(* Logix 5000 AddOnInstructionDefinition export EH_Smartec_CLD18_IOL; software revision 38.00 *)

TYPE EH_CommAOI_Data :
STRUCT
   Device_Comm_Error : BOOL;
   CommSuccess : BOOL;
   CommFailed : BOOL;
   CommTimeOut : BOOL;
   StateDone : BOOL;
   NewState : BOOL;
   OldState : SINT;
   PortSize : SINT;
   DevicePort : SINT;
   MaxState : SINT;
   State : SINT;
   VendorID : INT;
   DeviceID : DINT;
   CyclicData : INT[16];
   AcyclicData : DINT[8];
   ReplayIndex : INT;
   AOI_Diagnostic : DINT;
   ConnectionStatus : DINT;
   OutputData : INT[16];
END_STRUCT
END_TYPE

ADD_ON_INSTRUCTION EH_Smartec_CLD18_IOL   (* revision 1.0, vendor Endress+Hauser *)
// Smartec CLD18 Rev 1 IO-Link
VAR_IN_OUT
   DataToSend : INT[10]; {required}
   CommAOIBusy : DINT; {required}
   ActiveComPort : DINT; {required}
   DeviceAOISendRequest : DINT; {required}
   CommError : INT; {required}
   DeviceData : EH_CommAOI_Data; {required}
END_VAR
VAR_OUTPUT
   qVendor_ID : DINT; {access Read Only, visible}
   qDevice_ID : DINT; {access Read Only, visible}
END_VAR
VAR_INPUT
   iExecuteRisingEdge : BOOL; {visible}
   iSetSimulation : BOOL; {visible}
   iSetSimulationConductivity : REAL; {visible}
   iSetSimulationTemp : REAL; {visible}
   iParameterSet : SINT; {visible}
END_VAR
VAR_OUTPUT
   qConductivity : REAL; {visible}
   qTemperature : REAL; {visible}
   qCondensedStatus : USINT; {visible}
   qSSC1_1 : BOOL; {access Read Only, visible}
   qSSC1_2 : BOOL; {visible}
   qSSC2_1 : BOOL; {visible}
   qSSC2_2 : BOOL; {visible}
   qActiveParameterSet : BOOL; {visible}
   qSimulationActive : BOOL; {access Read Only, visible}
   qAOI_Diagnostic : DINT; {access Read Only, visible}
END_VAR
VAR_IN_OUT
   qActual_Diagnostics_String : STRING; {required}
END_VAR
VAR_OUTPUT
   qActual_Diagnostics_Code : DINT; {access Read Only, visible}
END_VAR
VAR_IN_OUT
   qLast_Diagnostics_String : STRING; {required}
END_VAR
VAR_OUTPUT
   qLast_Diagnostics_Code : DINT; {visible}
   qCommunicationBusy : DINT; {access Read Only, visible}
   qCommError : DINT; {access Read Only, visible}
   qDeviceConnectionError : BOOL; {access Read Only, visible}
END_VAR
VAR_INPUT
   DeviceID1 : DINT;
   qDevice_ID_select : INT;
END_VAR
VAR
   Calc_DID : DINT; {access None}
   Calc_VID : DINT; {access None}
   Cond_DINT : DINT; {access None}
   Temp_DINT : DINT; {access None}
   Calc_Cond : DINT; {access None}
   Cald_Temp : DINT; {access None}
   Calc_Temp : DINT; {access None}
   Calc_CondenStatus : DINT; {access None}
   CMD_Index : INT; {access None}
   CMD_Subindex : INT; {access None}
   CMD_ByteLength : INT; {access None}
   StateMin : INT; {access None}
   Trigger : BOOL; {access None}
   CMD_Rd : BOOL; {access None}
   CMD_Wr : BOOL; {access None}
   SimulationDINT : DINT; {access None}
   InputByteLength : DINT; {access None}
   oldCondStatus : USINT; {access None}
   ActiveAOI : BOOL; {access None}
   AOI_Prio : BOOL; {access None}
   firstTimeDone : BOOL; {access None}
   CondStatusChanged : BOOL; {access None}
   DeviceID : DINT; {access None}
   FALSE : BOOL; {access None}
   TRUE : BOOL := 1; {access None}
END_VAR

ROUTINE Logic   (* structured text *)
// CLD18 Communication via AL1323
   // =======================================================================
   // Endress+Hauser Digital Solutions
   // ©Copyright (2024) All Rights Reserved
   // =======================================================================
   // Name:                EH_Smartec_CLD18_IOL
   // Version:             1.0
   // Datum:               11.2025
   // Library:             01.01.00
   // Engineering:         Studio5000 V38.00.00
   // Author:              EH
   // =======================================================================
   
   
   qAOI_Diagnostic := DeviceData.AOI_Diagnostic;
   qCommunicationBusy := CommAOIBusy;
   DeviceID1 := 131329;
   StateMin := 0;
   DeviceData.MaxState := 8;
   
   if DeviceData.DevicePort = 0 or DeviceData.DeviceID <> DeviceID1 or DeviceData.ConnectionStatus <> 1 then
   
   	qVendor_ID	:= 0;
   	qDevice_ID	:= 0;
   	qConductivity	:= 0;
   	qTemperature	:= 0;
   	qCondensedStatus	:= 0;
   	qSSC1_1	:= 0;
   	qSSC1_2	:= 0;
   	qSSC2_1	:= 0;
   	qSSC2_2	:= 0;
   	qActiveParameterSet	:= 0;
   	qSimulationActive	:= 0;
   	qActual_Diagnostics_Code	:= 0;
   	qLast_Diagnostics_Code	:= 0;
   	qLast_Diagnostics_String	:= '';
   
   	if DeviceData.DevicePort = 0 then
   
   		qActual_Diagnostics_String	:= 'Device Port is Zero';
   		DeviceData.AOI_Diagnostic.1 := TRUE;
   
   	elsif DeviceData.ConnectionStatus <> 1 then
   
   		qActual_Diagnostics_String	:= 'No Device connected';
   		qDeviceConnectionError := TRUE;
   
   	elsif DeviceData.DeviceID <> DeviceID1 then
   
   		qActual_Diagnostics_String	:= 'Wrong DeviceID';
   		DeviceData.AOI_Diagnostic.2 := TRUE;
   		qVendor_ID := DeviceData.VendorID;
   		qDevice_ID := DeviceData.DeviceID;
   
   	end_if;
   
   else
   
   	if qActual_Diagnostics_Code = 0 then
   
   		qActual_Diagnostics_String	:= '--------';
   
   	end_if;
   
   	if qLast_Diagnostics_Code = 0 then
   
   		qLast_Diagnostics_String	:= '--------';
   
   	end_if;
   
   	DeviceData.AOI_Diagnostic.1 := FALSE;
   	qDeviceConnectionError := FALSE;
   	DeviceData.AOI_Diagnostic.2  := FALSE;
   
   end_if;
   
   
   if not DeviceData.AOI_Diagnostic.0
   	and not qDeviceConnectionError
   	and not DeviceData.AOI_Diagnostic.2
   	and DeviceData.DevicePort > 0 or ActiveAOI and qDeviceConnectionError then
   
   	//*********************************
   	//Vendor ID
   	//*********************************
   
   	qVendor_ID := DeviceData.VendorID;
   
   	//*********************************
   	//Device ID
   	//*********************************
   
   	qDevice_ID := DeviceData.DeviceID;
   
   	if DeviceData.DeviceID = DeviceID1 then
   
   		qDevice_ID_select :=1;
   
   	else
   
   		qDevice_ID_select := 0;
   
   	end_if;
   
   	case qDevice_ID_select of
   
   		1:
   
   		Calc_Cond 			:= 0+((DeviceData.DevicePort-1)*InputByteLength);  // Startwert 190 + Protnummer mal Datalength 32Byte
   		Calc_Temp 			:= 2+((DeviceData.DevicePort-1)*InputByteLength);  // Startwert 194 + Protnummer mal Datalength 32Byte
   		Calc_CondenStatus 	:= 4+((DeviceData.DevicePort-1)*InputByteLength); // Startwert 198 + Protnummer mal Datalength 32Byte
   
   		//*********************************
   		//Process Data Cond
   		//*********************************
   
   		Cond_DINT := DeviceData.CyclicData[Calc_Cond+1];
   		Cond_DINT.8 := DeviceData.CyclicData[Calc_Cond+1].8;
   		Cond_DINT.9 := DeviceData.CyclicData[Calc_Cond+1].9;
   		Cond_DINT.10 := DeviceData.CyclicData[Calc_Cond+1].10;
   		Cond_DINT.11 := DeviceData.CyclicData[Calc_Cond+1].11;
   		Cond_DINT.12 := DeviceData.CyclicData[Calc_Cond+1].12;
   		Cond_DINT.13 := DeviceData.CyclicData[Calc_Cond+1].13;
   		Cond_DINT.14 := DeviceData.CyclicData[Calc_Cond+1].14;
   		Cond_DINT.15 := DeviceData.CyclicData[Calc_Cond+1].15;
   		Cond_DINT.16 := DeviceData.CyclicData[Calc_Cond].0;
   		Cond_DINT.17 := DeviceData.CyclicData[Calc_Cond].1;
   		Cond_DINT.18 := DeviceData.CyclicData[Calc_Cond].2;
   		Cond_DINT.19 := DeviceData.CyclicData[Calc_Cond].3;
   		Cond_DINT.20 := DeviceData.CyclicData[Calc_Cond].4;
   		Cond_DINT.21 := DeviceData.CyclicData[Calc_Cond].5;
   		Cond_DINT.22 := DeviceData.CyclicData[Calc_Cond].6;
   		Cond_DINT.23 := DeviceData.CyclicData[Calc_Cond].7;
   		Cond_DINT.24 := DeviceData.CyclicData[Calc_Cond].8;
   		Cond_DINT.25 := DeviceData.CyclicData[Calc_Cond].9;
   		Cond_DINT.26 := DeviceData.CyclicData[Calc_Cond].10;
   		Cond_DINT.27 := DeviceData.CyclicData[Calc_Cond].11;
   		Cond_DINT.28 := DeviceData.CyclicData[Calc_Cond].12;
   		Cond_DINT.29 := DeviceData.CyclicData[Calc_Cond].13;
   		Cond_DINT.30 := DeviceData.CyclicData[Calc_Cond].14;
   		Cond_DINT.31 := DeviceData.CyclicData[Calc_Cond].15;
   
   		COP(Cond_DINT,qConductivity,1);
   
   		//*********************************
   		//Process Data Temp
   		//*********************************
   
   		Temp_DINT := DeviceData.CyclicData[Calc_Temp+1];
   		Temp_DINT.8 := DeviceData.CyclicData[Calc_Temp+1].8;
   		Temp_DINT.9 := DeviceData.CyclicData[Calc_Temp+1].9;
   		Temp_DINT.10 := DeviceData.CyclicData[Calc_Temp+1].10;
   		Temp_DINT.11 := DeviceData.CyclicData[Calc_Temp+1].11;
   		Temp_DINT.12 := DeviceData.CyclicData[Calc_Temp+1].12;
   		Temp_DINT.13 := DeviceData.CyclicData[Calc_Temp+1].13;
   		Temp_DINT.14 := DeviceData.CyclicData[Calc_Temp+1].14;
   		Temp_DINT.15 := DeviceData.CyclicData[Calc_Temp+1].15;
   		Temp_DINT.16 := DeviceData.CyclicData[Calc_Temp].0;
   		Temp_DINT.17 := DeviceData.CyclicData[Calc_Temp].1;
   		Temp_DINT.18 := DeviceData.CyclicData[Calc_Temp].2;
   		Temp_DINT.19 := DeviceData.CyclicData[Calc_Temp].3;
   		Temp_DINT.20 := DeviceData.CyclicData[Calc_Temp].4;
   		Temp_DINT.21 := DeviceData.CyclicData[Calc_Temp].5;
   		Temp_DINT.22 := DeviceData.CyclicData[Calc_Temp].6;
   		Temp_DINT.23 := DeviceData.CyclicData[Calc_Temp].7;
   		Temp_DINT.24 := DeviceData.CyclicData[Calc_Temp].8;
   		Temp_DINT.25 := DeviceData.CyclicData[Calc_Temp].9;
   		Temp_DINT.26 := DeviceData.CyclicData[Calc_Temp].10;
   		Temp_DINT.27 := DeviceData.CyclicData[Calc_Temp].11;
   		Temp_DINT.28 := DeviceData.CyclicData[Calc_Temp].12;
   		Temp_DINT.29 := DeviceData.CyclicData[Calc_Temp].13;
   		Temp_DINT.30 := DeviceData.CyclicData[Calc_Temp].14;
   		Temp_DINT.31 := DeviceData.CyclicData[Calc_Temp].15;
   
   		COP(Temp_DINT,qTemperature,1);
   
   		//*********************************
   		// Cond Status
   		//*********************************
   
   		qCondensedStatus.0 := DeviceData.CyclicData[Calc_CondenStatus].8;
   		qCondensedStatus.1 := DeviceData.CyclicData[Calc_CondenStatus].9;
   		qCondensedStatus.2 := DeviceData.CyclicData[Calc_CondenStatus].10;
   		qCondensedStatus.3 := DeviceData.CyclicData[Calc_CondenStatus].11;
   		qCondensedStatus.4 := DeviceData.CyclicData[Calc_CondenStatus].12;
   		qCondensedStatus.5 := DeviceData.CyclicData[Calc_CondenStatus].13;
   		qCondensedStatus.6 := DeviceData.CyclicData[Calc_CondenStatus].14;
   		qCondensedStatus.7 := DeviceData.CyclicData[Calc_CondenStatus].15;
   
   		//*********************************
   		//SSC Outputs
   		//*********************************
   
   		qSSC1_1 := DeviceData.CyclicData[Calc_CondenStatus].0;
   		qSSC1_2 := DeviceData.CyclicData[Calc_CondenStatus].1;
   		qSSC2_1 := DeviceData.CyclicData[Calc_CondenStatus].2;
   		qSSC2_2 := DeviceData.CyclicData[Calc_CondenStatus].3;
   
   		//*********************************
   		//Active Parameter Set
   		//*********************************
   
   		qActiveParameterSet := DeviceData.CyclicData[Calc_CondenStatus].4;
   
   		//*********************************
   		//CondenstStatus
   		//*********************************
   
   		qCondensedStatus.0 := DeviceData.CyclicData[Calc_CondenStatus].8;
   		qCondensedStatus.1 := DeviceData.CyclicData[Calc_CondenStatus].9;
   		qCondensedStatus.2 := DeviceData.CyclicData[Calc_CondenStatus].10;
   		qCondensedStatus.3 := DeviceData.CyclicData[Calc_CondenStatus].11;
   		qCondensedStatus.4 := DeviceData.CyclicData[Calc_CondenStatus].12;
   		qCondensedStatus.5 := DeviceData.CyclicData[Calc_CondenStatus].13;
   		qCondensedStatus.6 := DeviceData.CyclicData[Calc_CondenStatus].14;
   		qCondensedStatus.7 := DeviceData.CyclicData[Calc_CondenStatus].15;
   
   	end_case;
   
   	if  oldCondStatus = qCondensedStatus then
   
   		CondStatusChanged := 1;
   
   	else
   
   		CondStatusChanged := 0;
   
   	end_if;
   
   	//*********************************
   	// Checking for CommBlockBusy
   	//*********************************
   
   	if iExecuteRisingEdge and DeviceData.State = 0 and not ActiveAOI then
   		DeviceAOISendRequest.[DeviceData.DevicePort] := 1;
   
   	end_if;
   
   	if not CondStatusChanged and not ActiveAOI then
   		DeviceAOISendRequest.[DeviceData.DevicePort] := 1;
   
   	end_if;
   
   	if ActiveComPort = DeviceData.DevicePort then
   
   		AOI_Prio :=1;
   	else
   
   		AOI_Prio := 0;
   	end_if;
   
   
   	if CommAOIBusy = 1 and iExecuteRisingEdge and DeviceData.State = 0 and AOI_Prio and not ActiveAOI then
   
   		ActiveAOI := 1;
   
   	end_if;
   
   	if CommAOIBusy = 1 and not CondStatusChanged and (DeviceData.State = 0 or DeviceData.State = DeviceData.MaxState) and AOI_Prio and not ActiveAOI then
   
   		ActiveAOI := 1;
   
   	end_if;
   
   
   
   	qCommunicationBusy := CommAOIBusy;
   	qAOI_Diagnostic :=DeviceData.AOI_Diagnostic;
   
   
   	if  ActiveAOI and qDeviceConnectionError then
   
   		DeviceData.State := DeviceData.MaxState;
   
   	end_if;
   
   	//*********************************
   	// State machine
   	//*********************************
   
   	if ActiveAOI or DeviceData.State = DeviceData.MaxState then
   
   	case DeviceData.State of
   
   		//*********************************
   		0: // Idle
   		//*********************************
   
   			// Initializing
   			Trigger := 0;
   			CMD_Index := 0;
   			CMD_Subindex := 0;
   			CMD_Wr := 0;
   			CMD_Rd := 0;
   			CMD_ByteLength := 0;
   
   			if DeviceData.DevicePort = ActiveComPort then
   					DeviceData.CommSuccess := 0;
   					DeviceData.CommTimeOut := 0;
   					DeviceData.NewState := 1;
   					DeviceData.StateDone := 0;
   			end_if;
   
   			// Wait for trigger
   			if iExecuteRisingEdge and ActiveComPort = DeviceData.DevicePort then
   
   				DeviceData.AOI_Diagnostic := 0;
   				DeviceData.State := DeviceData.State + 1;
   
   			end_if;
   
   			if not CondStatusChanged then
   
   				DeviceData.State := DeviceData.MaxState - 2;
   				oldCondStatus := qCondensedStatus;
   
   			end_if;
   
   		//*********************************
   		1: // Simulation
   		//*********************************
   
   		    CMD_Index := 101;
   		    CMD_Subindex := 0;
   		    CMD_Wr := 1;
   			CMD_Rd := 0;
   		    CMD_ByteLength := 2;
   			DataToSend[6]:= 0;
   			DataToSend[7]:= 0;
   
   			if DeviceData.NewState then
   
   				DeviceData.StateDone := 1;
   
   			end_if;
   
   		    if iSetSimulation then
   
   		       DataToSend[6].8 := 1;
   
   		    else
   
   		        DataToSend[6].8 := 0;
   
   		    end_if;
   
   		    Trigger := 1;
   
   			if  DeviceData.CommSuccess and DeviceData.ReplayIndex = CMD_Index then
   
   				Trigger := 0;
   				DeviceData.OldState := DeviceData.State;
   		        DeviceData.State := DeviceData.State + 1;
   				DeviceData.CommSuccess := 0;
   				DeviceData.AcyclicData[0] := 0;
   				DeviceData.NewState := 1;
   
   			 elsif DeviceData.CommTimeOut then
   
   				DeviceData.AOI_Diagnostic.[DeviceData.State+7] := 1;
   				DeviceData.OldState := DeviceData.State;
   		        DeviceData.State := DeviceData.State + 1;
   				DeviceData.CommTimeOut := 0;
   				DeviceData.AcyclicData[0] := 0;
   				DeviceData.NewState := 1;
   
   		    end_if;
   
   		//*********************************
   		2: // Simulation - Value Cond
   		//*********************************
   
   		    CMD_Index := 102;
   		    CMD_Subindex := 0;
   		    CMD_Wr := 1;
   			CMD_Rd := 0;
   		    CMD_ByteLength := 4;
   
   			if DeviceData.NewState then
   
   				DeviceData.StateDone := 1;
   
   			end_if;
   
   			COP(iSetSimulationConductivity,SimulationDINT,1); // Kopiert den Inhalt des Real in ein DINT Format. Dabei wird nicht der eigentliche Realwert kopiert.
   
   			DataToSend[6].0 :=  SimulationDINT.24;
   			DataToSend[6].1 :=  SimulationDINT.25;
   			DataToSend[6].2 :=  SimulationDINT.26;
   			DataToSend[6].3 :=  SimulationDINT.27;
   			DataToSend[6].4 :=  SimulationDINT.28;
   			DataToSend[6].5 :=  SimulationDINT.29;
   			DataToSend[6].6 :=  SimulationDINT.30;
   			DataToSend[6].7 :=  SimulationDINT.31;
   			DataToSend[6].8 :=  SimulationDINT.16;
   			DataToSend[6].9 :=  SimulationDINT.17;
   			DataToSend[6].10 := SimulationDINT.18;
   			DataToSend[6].11 := SimulationDINT.19;
   			DataToSend[6].12 := SimulationDINT.20;
   			DataToSend[6].13 := SimulationDINT.21;
   			DataToSend[6].14 := SimulationDINT.22;
   			DataToSend[6].15 := SimulationDINT.23;
   			DataToSend[7].0  := SimulationDINT.8;
   			DataToSend[7].1  := SimulationDINT.9;
   			DataToSend[7].2  := SimulationDINT.10;
   			DataToSend[7].3  := SimulationDINT.11;
   			DataToSend[7].4  := SimulationDINT.12;
   			DataToSend[7].5  := SimulationDINT.13;
   			DataToSend[7].6  := SimulationDINT.14;
   			DataToSend[7].7  := SimulationDINT.15;
   			DataToSend[7].8  := SimulationDINT.0;
   			DataToSend[7].9  := SimulationDINT.1;
   			DataToSend[7].10 := SimulationDINT.2;
   			DataToSend[7].11 := SimulationDINT.3;
   			DataToSend[7].12 := SimulationDINT.4;
   			DataToSend[7].13 := SimulationDINT.5;
   			DataToSend[7].14 := SimulationDINT.6;
   			DataToSend[7].15 := SimulationDINT.7;
   			Trigger := 1;
   
   			if  DeviceData.CommSuccess and DeviceData.ReplayIndex = CMD_Index then
   
   				Trigger := 0;
   				DeviceData.OldState := DeviceData.State;
   		        DeviceData.State := DeviceData.State + 1;
   				DeviceData.CommSuccess := 0;
   				DeviceData.AcyclicData[0] := 0;
   				DeviceData.NewState := 1;
   
   			 elsif DeviceData.CommTimeOut then
   
   				DeviceData.AOI_Diagnostic.[DeviceData.State+7] := 1;
   				DeviceData.OldState := DeviceData.State;
   		        DeviceData.State := DeviceData.State + 1;
   				DeviceData.CommTimeOut := 0;
   				DeviceData.AcyclicData[0] := 0;
   				DeviceData.NewState := 1;
   
   		    end_if;
   
   		//*********************************
   		3: // Simulation - Value Temp
   		//*********************************
   
   		    CMD_Index := 103;
   		    CMD_Subindex := 0;
   		    CMD_Wr := 1;
   			CMD_Rd := 0;
   		    CMD_ByteLength := 4;
   
   			if DeviceData.NewState then
   
   				DeviceData.StateDone := 1;
   
   			end_if;
   
   			COP(iSetSimulationTemp,SimulationDINT,1); // Kopiert den Inhalt des Real in ein DINT Format. Dabei wird nicht der eigentliche Realwert kopiert.
   
   			DataToSend[6].0 :=  SimulationDINT.24;
   			DataToSend[6].1 :=  SimulationDINT.25;
   			DataToSend[6].2 :=  SimulationDINT.26;
   			DataToSend[6].3 :=  SimulationDINT.27;
   			DataToSend[6].4 :=  SimulationDINT.28;
   			DataToSend[6].5 :=  SimulationDINT.29;
   			DataToSend[6].6 :=  SimulationDINT.30;
   			DataToSend[6].7 :=  SimulationDINT.31;
   			DataToSend[6].8 :=  SimulationDINT.16;
   			DataToSend[6].9 :=  SimulationDINT.17;
   			DataToSend[6].10 := SimulationDINT.18;
   			DataToSend[6].11 := SimulationDINT.19;
   			DataToSend[6].12 := SimulationDINT.20;
   			DataToSend[6].13 := SimulationDINT.21;
   			DataToSend[6].14 := SimulationDINT.22;
   			DataToSend[6].15 := SimulationDINT.23;
   			DataToSend[7].0  := SimulationDINT.8;
   			DataToSend[7].1  := SimulationDINT.9;
   			DataToSend[7].2  := SimulationDINT.10;
   			DataToSend[7].3  := SimulationDINT.11;
   			DataToSend[7].4  := SimulationDINT.12;
   			DataToSend[7].5  := SimulationDINT.13;
   			DataToSend[7].6  := SimulationDINT.14;
   			DataToSend[7].7  := SimulationDINT.15;
   			DataToSend[7].8  := SimulationDINT.0;
   			DataToSend[7].9  := SimulationDINT.1;
   			DataToSend[7].10 := SimulationDINT.2;
   			DataToSend[7].11 := SimulationDINT.3;
   			DataToSend[7].12 := SimulationDINT.4;
   			DataToSend[7].13 := SimulationDINT.5;
   			DataToSend[7].14 := SimulationDINT.6;
   			DataToSend[7].15 := SimulationDINT.7;
   			Trigger := 1;
   
   			if  DeviceData.CommSuccess and DeviceData.ReplayIndex = CMD_Index then
   
   				Trigger := 0;
   				DeviceData.OldState := DeviceData.State;
   		        DeviceData.State := DeviceData.State + 1;
   				DeviceData.CommSuccess := 0;
   				DeviceData.AcyclicData[0] := 0;
   				DeviceData.NewState := 1;
   
   			 elsif DeviceData.CommTimeOut then
   
   				DeviceData.AOI_Diagnostic.[DeviceData.State+7] := 1;
   				DeviceData.OldState := DeviceData.State;
   		        DeviceData.State := DeviceData.State + 1;
   				DeviceData.CommTimeOut := 0;
   				DeviceData.AcyclicData[0] := 0;
   				DeviceData.NewState := 1;
   
   		    end_if;
   
   		//*********************************
   		4: // Simulation - Value ParameterSet
   		//*********************************
   
   		    CMD_Index := 112;
   		    CMD_Subindex := 0;
   		    CMD_Wr := 1;
   			CMD_Rd := 0;
   		    CMD_ByteLength := 1;
   			DataToSend[6]:= 0;
   			DataToSend[7]:= 0;
   			Trigger := 1;
   
   			if DeviceData.NewState then
   
   				DeviceData.StateDone := 1;
   
   			end_if;
   
   			if iParameterSet = 1 then
   
   		       DataToSend[6] := 0;
   
   		    elsif iParameterSet = 2 then
   
   		        DataToSend[6] := 1;
   
   		    end_if;
   
   			if  DeviceData.CommSuccess and DeviceData.ReplayIndex = CMD_Index then
   
   				Trigger := 0;
   				DeviceData.OldState := DeviceData.State;
   		        DeviceData.State := DeviceData.State + 1;
   				DeviceData.CommSuccess := 0;
   				DeviceData.AcyclicData[0] := 0;
   				DeviceData.NewState := 1;
   
   			 elsif DeviceData.CommTimeOut then
   
   				DeviceData.AOI_Diagnostic.[DeviceData.State+7] := 1;
   				DeviceData.OldState := DeviceData.State;
   		        DeviceData.State := DeviceData.State + 1;
   				DeviceData.CommTimeOut := 0;
   				DeviceData.AcyclicData[0] := 0;
   				DeviceData.NewState := 1;
   
   		    end_if;
   
   		//*********************************
   		5: // Simulation - SimulationActive
   		//*********************************
   
   		    CMD_Index := 101;
   		    CMD_Subindex := 0;
   		    CMD_Wr := 0;
   			CMD_Rd := 1;
   		    CMD_ByteLength := 0;
   			Trigger := 1;
   
   			if DeviceData.NewState then
   
   				DeviceData.StateDone := 1;
   
   			end_if;
   
   			if  DeviceData.CommSuccess and DeviceData.ReplayIndex = CMD_Index then
   
   				qSimulationActive := DeviceData.AcyclicData[0].0;
   
   				Trigger := 0;
   				DeviceData.OldState := DeviceData.State;
   		        DeviceData.State := DeviceData.State + 1;
   				DeviceData.CommSuccess := 0;
   				DeviceData.AcyclicData[0] := 0;
   				DeviceData.NewState := 1;
   
   			 elsif DeviceData.CommTimeOut then
   
   				DeviceData.AOI_Diagnostic.[DeviceData.State+7] := 1;
   				DeviceData.OldState := DeviceData.State;
   		        DeviceData.State := DeviceData.State + 1;
   				DeviceData.CommTimeOut := 0;
   				DeviceData.AcyclicData[0] := 0;
   				DeviceData.NewState := 1;
   
   		    end_if;
   
   		//*********************************
   		6: // Actual Diagnostic
   		//*********************************
   
   		    CMD_Index := 260;
   		    CMD_Subindex := 0;
   		    CMD_Wr := 0;
   			CMD_Rd := 1;
   		    Trigger := 1;
   			if DeviceData.NewState then
   			DeviceData.StateDone := 1;
   			end_if;
   
   			if  DeviceData.CommSuccess and DeviceData.ReplayIndex = CMD_Index then
   
   				qActual_Diagnostics_Code	:= DeviceData.AcyclicData[0];
   
   				case qActual_Diagnostics_Code of
   
   		            0:
   		                qActual_Diagnostics_String := 'System ok';
   		            1:
   		                qActual_Diagnostics_String := 'no communication';
   		            22:
   		                qActual_Diagnostics_String := 'F022 Temperature sensor is defective';
   		            61:
   		                qActual_Diagnostics_String := 'F061 Sensor electronics defective';
   		            100:
   		                qActual_Diagnostics_String := 'F100 Sensor not communicating, not connected';
   		            130:
   		                qActual_Diagnostics_String := 'F130 Sensor check, no conductivity displayed';
   		            152:
   		                qActual_Diagnostics_String := 'F152 Sensor data No calibration data available';
   		            241:
   		                qActual_Diagnostics_String := 'F241 Unspecific software error';
   		            243:
   		                qActual_Diagnostics_String := 'F243 Unspecific hardware error';
   		            419:
   		                qActual_Diagnostics_String := 'F419 Back to box command is executed';
   		            904:
   		                qActual_Diagnostics_String := 'F904 Process check system alarm';
   		            107:
   		                qActual_Diagnostics_String := 'C107 Sensor calibration is active';
   		            216:
   		                qActual_Diagnostics_String := 'C216 Hold function is active';
   		            848:
   		                qActual_Diagnostics_String := 'C848 Simulation active';
   		            144:
   		                qActual_Diagnostics_String := 'S144 Conductivity outside measuring range';
   		            146:
   		                qActual_Diagnostics_String := 'S146 Temperature outside measuring range';
   		            460:
   		            	qActual_Diagnostics_String := 'S46 0Output limit value undershot';
   		        	461:
   			            qActual_Diagnostics_String := 'S461 Output limit value overshot';
   		        	500:
   		        	    qActual_Diagnostics_String := 'M500 Sensor calibration aborted';
   					else
   						qActual_Diagnostics_String := 'Error Code unknown';
   
   		 		end_case;
   
   				Trigger := 0;
   				DeviceData.OldState := DeviceData.State;
   		        DeviceData.State := DeviceData.State + 1;
   				DeviceData.CommSuccess := 0;
   				DeviceData.AcyclicData[0] := 0;
   				DeviceData.NewState := 1;
   
   			 elsif DeviceData.CommTimeOut then
   
   				DeviceData.AOI_Diagnostic.[DeviceData.State+7] := 1;
   				DeviceData.OldState := DeviceData.State;
   		        DeviceData.State := DeviceData.State + 1;
   				DeviceData.CommTimeOut := 0;
   				DeviceData.AcyclicData[0] := 0;
   				DeviceData.NewState := 1;
   
   		    end_if;
   
   		//*********************************
   		7: // Last Diagnostic
   		//*********************************
   
   		    CMD_Index := 261;
   			CMD_Subindex := 0;
   		    CMD_Wr := 0;
   			CMD_Rd := 1;
   		    Trigger := 1;
   
   			if DeviceData.NewState then
   
   				DeviceData.StateDone := 1;
   
   			end_if;
   
   			if  DeviceData.CommSuccess and DeviceData.ReplayIndex = CMD_Index then
   
   				qLast_Diagnostics_Code	:= DeviceData.AcyclicData[0];
   
   				case qLast_Diagnostics_Code of
   
   					0:
   		                qLast_Diagnostics_String := 'System ok';
   		            1:
   		                qLast_Diagnostics_String := 'no communication';
   		            22:
   		                qLast_Diagnostics_String := 'F022 Temperature sensor is defective';
   		            61:
   		                qLast_Diagnostics_String := 'F061 Sensor electronics defective';
   		            100:
   		                qLast_Diagnostics_String := 'F100 Sensor not communicating, not connected';
   		            130:
   		                qLast_Diagnostics_String := 'F130 Sensor check, no conductivity displayed';
   		            152:
   		                qLast_Diagnostics_String := 'F152 Sensor data No calibration data available';
   		            241:
   		                qLast_Diagnostics_String := 'F241 Unspecific software error';
   		            243:
   		                qLast_Diagnostics_String := 'F243 Unspecific hardware error';
   		            419:
   		                qLast_Diagnostics_String := 'F419 Back to box command is executed';
   					904:
   		                qLast_Diagnostics_String := 'F904 Process check system alarm';
   		            107:
   		                qLast_Diagnostics_String := 'C107 Sensor calibration is active';
   		            216:
   		                qLast_Diagnostics_String := 'C216 Hold function is active';
   		            848:
   		                qLast_Diagnostics_String := 'C848 Simulation active';
   		            144:
   		                qLast_Diagnostics_String := 'S144 Conductivity outside measuring range';
   		            146:
   		                qLast_Diagnostics_String := 'S146 Temperature outside measuring range';
   		            460:
   		            	qLast_Diagnostics_String := 'S460 Output limit value undershot';
   		        	461:
   			            qLast_Diagnostics_String := 'S461 Output limit value overshot';
   		        	500:
   		        	    qLast_Diagnostics_String := 'M500 Sensor calibration aborted';
   					else
   						qLast_Diagnostics_String := 'Error Code unknown';
   
   		 		end_case;
   
   				Trigger := 0;
   				DeviceData.OldState := DeviceData.State;
   		        DeviceData.State := DeviceData.State + 1;
   				DeviceData.CommSuccess := 0;
   				DeviceData.AcyclicData[0] := 0;
   				DeviceData.NewState := 1;
   
   			 elsif DeviceData.CommTimeOut then
   
   				DeviceData.AOI_Diagnostic.[DeviceData.State+7] := 1;
   				DeviceData.OldState := DeviceData.State;
   		        DeviceData.State := DeviceData.State + 1;
   				DeviceData.CommTimeOut := 0;
   				DeviceData.AcyclicData[0] := 0;
   				DeviceData.NewState := 1;
   
   		    end_if;
   
   		//*********************************
   		8: // Trigger guard
   		//*********************************
   
   			if not firstTimeDone then
   
   				CommAOIBusy := 0;
   				firstTimeDone := 1;
   				DeviceAOISendRequest.[DeviceData.DevicePort] := 0;
   				ActiveComPort := 0;
   				ActiveAOI := 0;
   				DataToSend[0] := 0;
   				DataToSend[1] := 0;
   				DataToSend[2] := 0;
   				DataToSend[3] := 0;
   				DataToSend[4] := 0;
   				DataToSend[5] := 0;
    				DataToSend[6] := 0;
   				DataToSend[7] := 0;
   				DataToSend[8] := 0;
   				DataToSend[9] := 0;
   				DeviceData.StateDone := 0;
   
   			end_if;
   
   			if DeviceData.State =  DeviceData.MaxState AND NOT iExecuteRisingEdge then
   
   				DeviceData.State := 0;
   				DeviceData.OldState := DeviceData.State;
   				firstTimeDone := 0;
   
   			end_if;
   
   	end_case;
   
   	end_if;
   
   
   	//*************************
   	// Execution Area
   	//*************************
   
   	if DeviceData.State > StateMin and DeviceData.State < DeviceData.MaxState then
   
   
   	DataToSend[2] := DeviceData.DevicePort;
   	DataToSend[3] := CMD_Index;
   	DataToSend[4] := CMD_Subindex;
   	DataToSend[5].0 := CMD_Rd;
   	DataToSend[5].1 := CMD_Wr;
   	DataToSend[5].8 := CMD_ByteLength.0;  // Bits für die Länge
   	DataToSend[5].9 := CMD_ByteLength.1;
   	DataToSend[5].10 := CMD_ByteLength.2;
   	DataToSend[5].11 := CMD_ByteLength.3;
   	DataToSend[5].12 := CMD_ByteLength.4;
   	DataToSend[5].13 := CMD_ByteLength.5;
   	DataToSend[5].14 := CMD_ByteLength.6;
   	DataToSend[5].15 := CMD_ByteLength.7;
   
   	DataToSend[5].7 := Trigger;
   
   	qCommError := CommError;
   
   	end_if;
   
   end_if;
END_ROUTINE
END_ADD_ON_INSTRUCTION
